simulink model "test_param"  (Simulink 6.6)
settings: Solver=ode45  StartTime=0.0  StopTime=10.0  RelTol=1e-3
libraries: sltpda x3

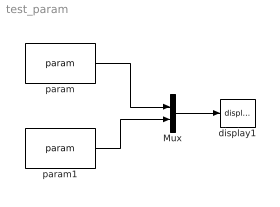
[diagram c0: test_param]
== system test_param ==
  Mux : Mux  Inputs=2
  display1 : sltpda/AO class/display  Tag=display  SystemSampleTime=-1
  param : sltpda/AO class/param  SystemSampleTime=-1  key=a  value=1
  param1 : sltpda/AO class/param  SystemSampleTime=-1  key=b  value=2
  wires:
  param/1 -> Mux/1
  param1/1 -> Mux/2
  Mux/1 -> display1/1
